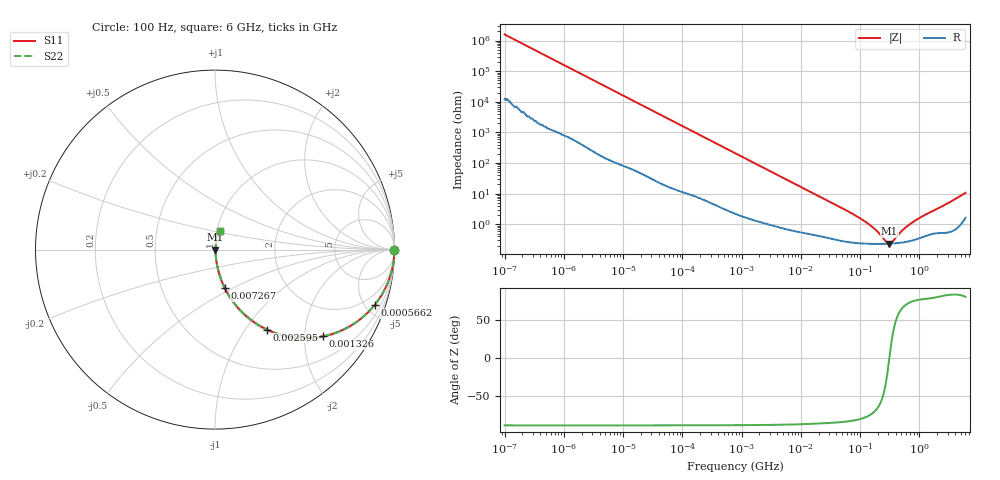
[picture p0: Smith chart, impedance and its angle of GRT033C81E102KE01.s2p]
!Murata Part Number: GRT033C81E102KE01
!These Parameters are Measured in Series Mode Connection
!Data Generated on Jun 19, 2026
!  o--ll--o
!Port1  Port2
!  o------o
!Operation Temp=25[degC], DC Bias Voltage=0[V]
!Freq. Start=100[Hz] Stop=6[GHz] 401[Steps]
# Hz S RI R 50
!Freq.(Hz) S11(Real) S11(Imag) S21(Real) S21(Imag) S12(Real) S12(Imag) S22(Real) S22(Imag)
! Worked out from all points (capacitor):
!   401 points, 100 Hz to 6 GHz, reference 50 ohm
!   read as one part in series: C = 1 nF near 109 Hz
!   lowest |Z| = 233 mohm at 312.4 MHz (marker M1)
!   series resonance near 312.5 MHz, so ESL is about 260 pH
!   S11 on the Smith chart (normalised r, x): 100 Hz: open; 566.2 kHz: 1.06, -5.76; 1.326 MHz: 1.03, -2.47; 2.595 MHz: 1.02, -1.27; 7.267 MHz: 1.01, -0.46; 6 GHz: 1.03, +0.21
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100  1 -6.32e-05  5e-07 6.32e-05  5e-07 6.32e-05  1 -6.32e-05
171  1 -0.000108  7e-07 0.000108  7e-07 0.000108  1 -0.000108
2008  1 -0.00126  7.9e-06 0.00126  7.9e-06 0.00126  1 -0.00126
40335  0.9992 -0.025  0.000769 0.025  0.000769 0.025  0.9992 -0.025
184852  0.9862 -0.1123  0.0138 0.1123  0.0138 0.1123  0.9862 -0.1123
566185  0.8902 -0.3078  0.1098 0.3078  0.1098 0.3078  0.8902 -0.3078
774597  0.814 -0.3839  0.186 0.3839  0.186 0.3839  0.814 -0.3839
1325623  0.6033 -0.4831  0.3967 0.4831  0.3967 0.4831  0.6033 -0.4831
1813585  0.4512 -0.4907  0.5488 0.4907  0.5488 0.4907  0.4512 -0.4907
2594782  0.2901 -0.4457  0.7099 0.4457  0.7099 0.4457  0.2901 -0.4457
4246196  0.1366 -0.3334  0.8634 0.3334  0.8634 0.3334  0.1366 -0.3334
7266822  0.0549 -0.2146  0.9451 0.2146  0.9451 0.2146  0.0549 -0.2146
1.555665e7  0.0159 -0.1054  0.9841 0.1054  0.9841 0.1054  0.0159 -0.1054
5.449875e7  0.00366 -0.0304  0.9963 0.0304  0.9963 0.0304  0.00366 -0.0304
1.115611e8  0.00253 -0.0135  0.9975 0.0135  0.9975 0.0135  0.00253 -0.0135
1.669249e8  0.00234 -0.00738  0.9977 0.00738  0.9977 0.00738  0.00234 -0.00738
2.731619e8  0.0023 -0.00149  0.9977 0.00149  0.9977 0.00149  0.0023 -0.00149
3.124326e8  0.00232 -3.7e-06  0.9977 3.7e-06  0.9977 3.7e-06  0.00232 -3.7e-06
3.573489e8  0.00236 0.00148  0.9976 -0.00148  0.9976 -0.00148  0.00236 0.00148
5.59173e8  0.00264 0.00674  0.9974 -0.00674  0.9974 -0.00674  0.00264 0.00674
8.000355e8  0.00316 0.0118  0.9968 -0.0118  0.9968 -0.0118  0.00316 0.0118
6e9  0.0264 0.1009  0.9736 -0.1009  0.9736 -0.1009  0.0264 0.1009
